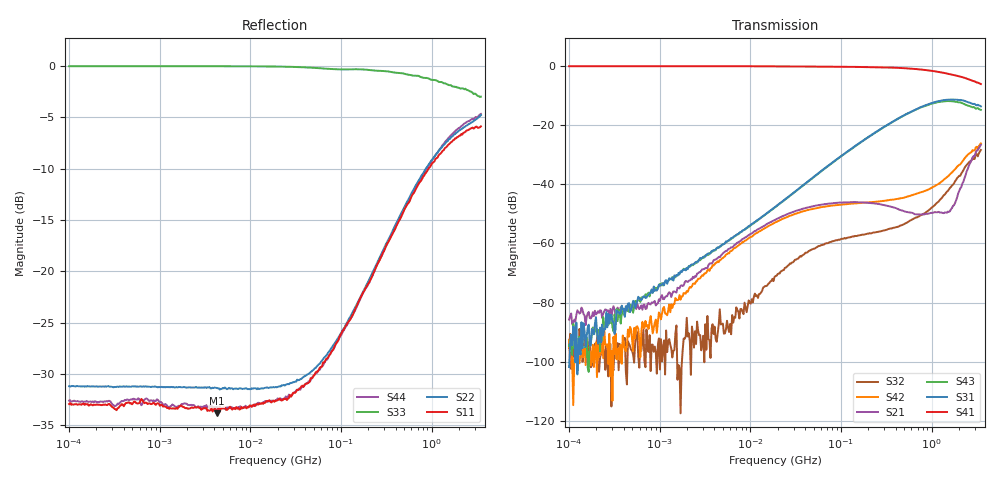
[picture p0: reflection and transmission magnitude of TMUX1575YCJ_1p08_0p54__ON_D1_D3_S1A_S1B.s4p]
!Keysight Technologies,E5080A,MY55200740,A.12.60.03
!Date: Wednesday, July 22, 2020 12:05:52
!Correction: S11(Full 4 Port(1,2,3,4))
!S12(Full 4 Port(1,2,3,4))
!S13(Full 4 Port(1,2,3,4))
!S14(Full 4 Port(1,2,3,4))
!S21(Full 4 Port(1,2,3,4))
!S22(Full 4 Port(1,2,3,4))
!S23(Full 4 Port(1,2,3,4))
!S24(Full 4 Port(1,2,3,4))
!S31(Full 4 Port(1,2,3,4))
!S32(Full 4 Port(1,2,3,4))
!S33(Full 4 Port(1,2,3,4))
!S34(Full 4 Port(1,2,3,4))
!S41(Full 4 Port(1,2,3,4))
!S42(Full 4 Port(1,2,3,4))
!S43(Full 4 Port(1,2,3,4))
!S44(Full 4 Port(1,2,3,4))
!S4P File: Measurements: <S11,S12,S13,S14>,
!<S21,S22,S23,S24>,
!<S31,S32,S33,S34>,
!<S41,S42,S43,S44>:Log Frequency Sweep
# Hz S  dB  R 50
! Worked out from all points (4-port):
!   400 points, 100 kHz to 3.5 GHz, reference 50 ohm
!   strongest paths, dB at 100 kHz, 1.377 MHz, 18.96 MHz, 261 MHz, 3.5 GHz:
!     S41: -0.2, -0.2, -0.2, -0.5, -6.2
!     S31: -101.7, -71.6, -47.6, -21.8, -13.8
!     S43: -94.6, -71.4, -47.7, -21.9, -14.9
!     S21: -85.7, -76.9, -52.0, -46.7, -26.7
!     S42: -92.6, -81.8, -52.8, -45.8, -26.2
!     S32: -95.3, -98.5, -71.0, -56.0, -28.5
!   lowest |S11| = -33.8 dB at 4.252 MHz (marker M1), VSWR 1.04, Z = 52 - j0.51 ohm
!   |S11| at or under -10 dB: start of sweep to 923.4 MHz
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100000  -32.94 5.6  -91.17 67.0  -104.67 46.1  -0.20 -0.0
        -85.70 163.0  -31.21 1.6  -100.96 -122.0  -84.71 -160.1
        -101.74 28.4  -95.30 -43.7  0.00 -0.0  -91.81 18.3
        -0.20 -0.0  -92.56 122.1  -94.55 120.6  -32.61 5.8
1306432  -33.35 -6.7  -80.90 111.0  -71.84 92.5  -0.19 -0.1
         -76.83 -178.7  -31.30 -3.2  -106.40 122.6  -76.89 -175.4
         -71.99 95.1  -94.11 42.0  0.00 -0.1  -71.94 92.2
         -0.19 -0.1  -83.26 112.4  -71.92 91.2  -33.17 -7.0
4251829  -33.85 -14.0  -65.52 104.6  -61.63 95.7  -0.20 -0.3
         -65.15 133.8  -31.38 -10.1  -91.03 57.5  -65.26 139.2
         -61.65 95.2  -93.20 125.0  -0.00 -0.3  -61.65 92.2
         -0.20 -0.3  -66.48 107.8  -61.55 94.9  -33.22 -12.4
1.06458e7  -33.07 -33.3  -56.49 83.0  -53.32 97.9  -0.22 -0.7
           -56.37 94.2  -31.46 -23.3  -78.47 113.3  -57.21 96.2
           -53.25 98.3  -79.94 105.9  -0.01 -0.9  -53.39 98.3
           -0.22 -0.7  -57.43 83.0  -53.36 98.2  -33.14 -31.7
5.554726e7  -29.78 -77.3  -47.14 33.3  -36.46 99.1  -0.34 -2.3
            -47.10 35.7  -29.17 -70.1  -61.20 62.9  -47.98 27.3
            -36.45 99.2  -61.10 61.9  -0.18 -4.6  -36.56 99.8
            -0.34 -2.3  -47.97 24.9  -36.55 99.7  -29.74 -79.1
1.552459e9  -7.62 -133.1  -49.39 105.5  -11.48 15.0  -2.81 -32.4
            -49.39 105.6  -7.10 -128.3  -41.79 -89.9  -37.11 -116.3
            -11.48 15.1  -41.80 -89.9  -1.84 -76.4  -11.98 31.3
            -2.79 -32.4  -37.11 -116.4  -11.97 31.1  -6.95 -121.7
3.5e9  -5.87 -157.9  -26.77 143.1  -13.79 -15.3  -6.25 -50.9
       -26.74 143.0  -4.76 -141.8  -28.48 176.3  -26.28 173.5
       -13.75 -15.4  -28.47 176.0  -2.97 -112.4  -14.93 37.9
       -6.21 -51.0  -26.24 173.6  -14.94 37.9  -4.66 -144.0
